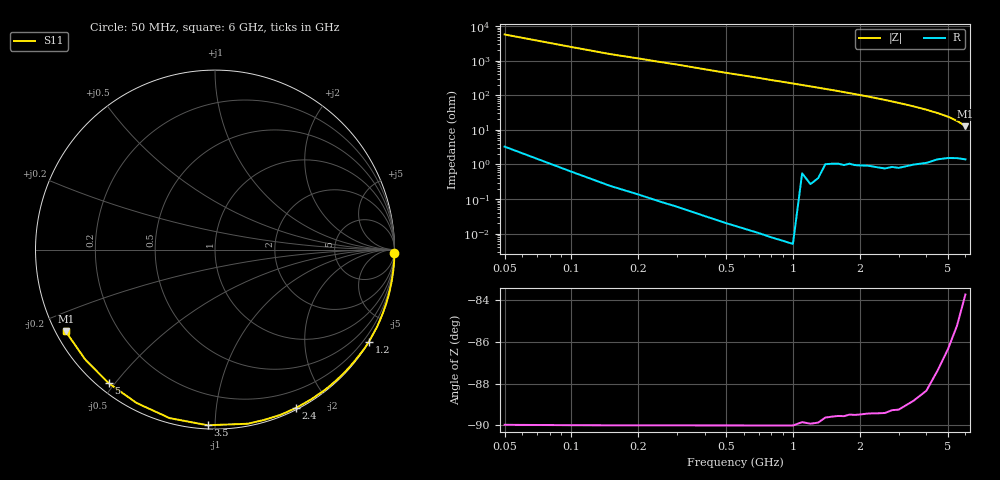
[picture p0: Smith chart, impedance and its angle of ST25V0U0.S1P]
! SIEMENS Discrete & RF Semiconductors
! BA892
! Si PIN Diode in SCD-80
! VR = 25 V
! S-Parameters:  September  1997
# GHz  S  MA  R  50
!  f  S11
! GHz  MAG  ANG
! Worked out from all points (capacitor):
!   34 points, 50 MHz to 6 GHz, reference 50 ohm
!   read as one part to ground: C = 639 fF near 50 MHz
!   lowest |Z| = 12.9 ohm at 6 GHz (marker M1)
!   S11 on the Smith chart (normalised r, x): 50 MHz: open; 1.2 GHz: 0.01, -3.62; 2.4 GHz: 0.02, -1.63; 3.5 GHz: 0.02, -0.96; 5 GHz: 0.03, -0.48; 6 GHz: 0.03, -0.26
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0.05  1 -1.0
0.15  1 -3.7
0.2  1 -4.9
0.3  1 -7.4
0.4  1 -10.1
0.5  1 -12.8
0.6  1 -15.3
0.7  1 -17.8
0.8  1 -20.6
1  1 -25.7
1.2  0.9992 -30.9
1.3  0.9987 -33.5
1.4  0.9961 -36.2
1.5  0.9954 -38.7
1.6  0.9947 -41.4
1.8  0.9934 -46.8
2  0.9928 -52.1
2.2  0.9916 -57.5
2.4  0.991 -63.0
2.6  0.9903 -68.5
2.8  0.9878 -74.0
3  0.987 -79.4
3.5  0.9796 -92.4
4  0.9723 -105.1
4.5  0.9597 -117.1
5  0.9513 -128.5
5.5  0.9475 -139.9
6  0.9486 -151.3
